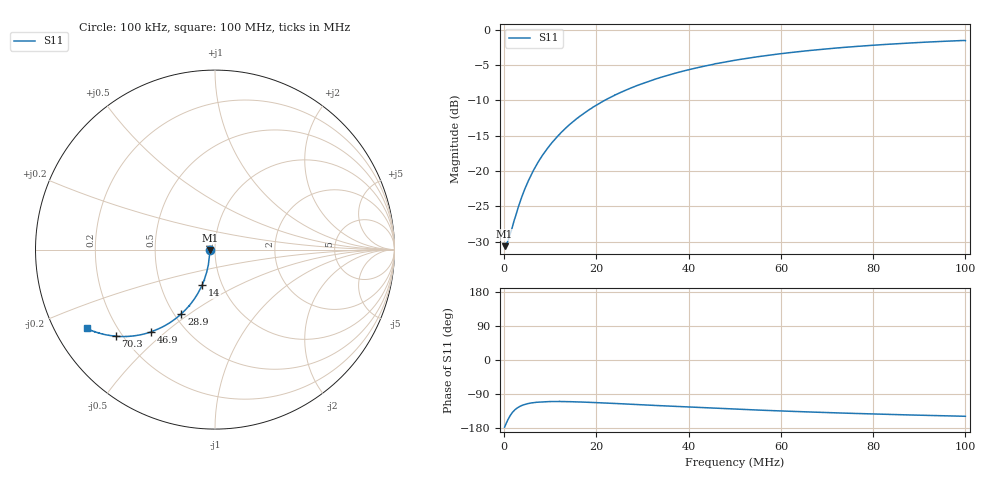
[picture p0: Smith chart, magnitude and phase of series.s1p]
# Hz S RI R 50.0
! written by SimSmith version 18.3h
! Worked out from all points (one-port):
!   1000 points, 100 kHz to 100 MHz, reference 50 ohm
!   lowest |S11| = -30.7 dB at 100 kHz (marker M1), VSWR 1.06, Z = 47.2 - j0.139 ohm
!   |S11| at or under -10 dB: start of sweep to 21.8 MHz
!   S11 on the Smith chart (normalised r, x): 100 kHz: 0.94, -0.00; 14 MHz: 0.80, -0.33; 28.9 MHz: 0.55, -0.47; 46.9 MHz: 0.32, -0.45; 70.3 MHz: 0.18, -0.37; 100 MHz: 0.10, -0.28
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100000  -0.0293 -0.00147
500000  -0.0295 -0.00751
900000  -0.0296 -0.0134
1400000  -0.0299 -0.021
3100000  -0.0316 -0.0461
3700000  -0.0326 -0.0547
4900000  -0.035 -0.0722
6100000  -0.0379 -0.0894
7400000  -0.0418 -0.1079
9000000  -0.0475 -0.1305
1.08e7  -0.0553 -0.1551
1.26e7  -0.064 -0.1793
1.4e7  -0.0717 -0.1976
1.63e7  -0.086 -0.2265
1.9e7  -0.1044 -0.2585
2.21e7  -0.1281 -0.293
2.51e7  -0.153 -0.3231
2.89e7  -0.1867 -0.3571
3.32e7  -0.227 -0.39
3.76e7  -0.2692 -0.4178
4.69e7  -0.3577 -0.459
5.01e7  -0.3877 -0.4681
5.66e7  -0.445 -0.4797
6.26e7  -0.4942 -0.484
7.03e7  -0.5515 -0.4824
7.51e7  -0.5843 -0.4787
8.76e7  -0.6578 -0.4617
1e8  -0.7126 -0.4354
